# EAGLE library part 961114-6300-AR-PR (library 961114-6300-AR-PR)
Headers & Wire Housings 14P STR SMT SR GOLD 5.3MM MATING PIN Source: Datasheet
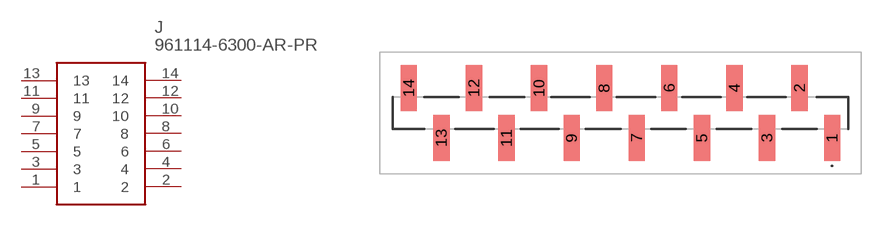
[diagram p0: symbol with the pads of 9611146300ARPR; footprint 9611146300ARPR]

Designator prefix J

## 961114-6300-AR-PR (Description: Headers & Wire Housings 14P STR SMT SR GOLD 5.3MM MATING PIN; Height: 9.6mm; Manufacturer_Name: 3M; Manufacturer_Part_Number: 961114-6300-AR-PR; Mouser_Part_Number: 517-9611146300ARPR; Mouser_Price-Stock: https://www.mouser.com/Search/Refine.aspx?Keyword=517-9611146300ARPR)  [9611146300ARPR]
1  1
2  2
3  3
4  4
5  5
6  6
7  7
8  8
9  9
10  10
11  11
12  12
13  13
14  14

## Footprint 9611146300ARPR (pad centres in mm)
961114-6300-AR-PR-4
smd 1.27 x 3.6: 1 16.51,-1.95; 2 13.97,1.95; 3 11.43,-1.95; 4 8.89,1.95; 5 6.35,-1.95; 6 3.81,1.95; 7 1.27,-1.95; 8 -1.27,1.95; 9 -3.81,-1.95; 10 -6.35,1.95; 11 -8.89,-1.95; 12 -11.43,1.95; 13 -13.97,-1.95; 14 -16.51,1.95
